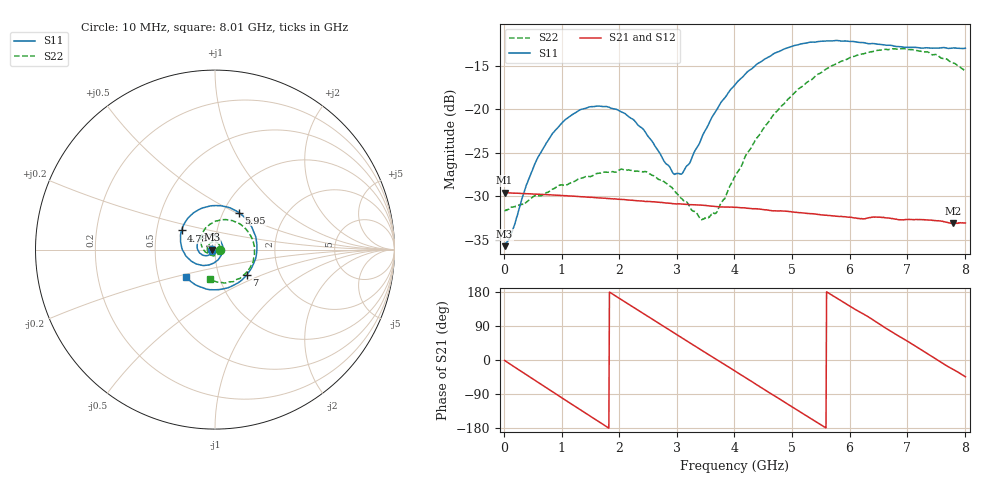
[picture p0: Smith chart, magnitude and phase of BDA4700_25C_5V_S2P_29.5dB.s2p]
!Agilent Technologies,E5071B,MY42404982,A.09.10
!Date: Mon Oct 20 13:41:26 2025
!Data & Calibration Information:
!Freq	S11:SOLT2(ON)	S21:SOLT2(ON)	S12:SOLT2(ON)	S22:SOLT2(ON)
# Hz S RI R 50
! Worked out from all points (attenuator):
!   801 points, 10 MHz to 8.01 GHz, reference 50 ohm
!   highest |S21| = -29.57 dB at 10 MHz (marker M1); lowest = -33.1 dB at 7.8 GHz (marker M2)
!   lowest |S11| = -35.7 dB at 10 MHz (marker M3), VSWR 1.03, Z = 48.4 - j0.113 ohm
!   |S11| at or under -10 dB: start of sweep to end of sweep
!   |S22| runs from -32.7 to -13.0 dB; largest |S21 - S12| = 0.0003
!   S11 on the Smith chart (normalised r, x): 10 MHz: 0.97, -0.00; 4.78 GHz: 0.67, +0.15; 5.95 GHz: 1.19, +0.52; 7 GHz: 1.37, -0.40; 8.01 GHz: 0.69, -0.22
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1e7  -0.0163 -0.00117  0.0332 -0.000676  0.0332 -0.000717  0.0262 -0.0008
1.4e8  -0.0176 -0.00937  0.032 -0.00815  0.032 -0.00817  0.0266 -0.00674
3.9e8  -0.0268 -0.0253  0.0254 -0.0207  0.0254 -0.0207  0.021 -0.0204
6.2e8  -0.0435 -0.0337  0.0153 -0.0287  0.0152 -0.0287  0.0115 -0.0297
1.01e9  -0.0804 -0.0235  -0.00579 -0.0315  -0.00583 -0.0314  -0.0152 -0.0335
1.35e9  -0.0995 0.00964  -0.0218 -0.0227  -0.0218 -0.0227  -0.036 -0.0179
2.08e9  -0.047 0.0827  -0.0275 0.0128  -0.0274 0.0128  -0.0299 0.0335
2.68e9  0.0313 0.0482  -0.00364 0.029  -0.00367 0.029  0.0126 0.0375
2.94e9  0.0421 0.00773  0.00866 0.0274  0.0087 0.0274  0.025 0.0242
3.09e9  0.0387 -0.0179  0.0151 0.0242  0.015 0.0243  0.0278 0.0126
3.42e9  0.00371 -0.0669  0.0251 0.0127  0.0251 0.0127  0.0198 -0.0121
3.54e9  -0.0162 -0.0787  0.0269 0.00737  0.027 0.00736  0.013 -0.02
3.7e9  -0.0492 -0.087  0.0276 0.000138  0.0276 4.01e-05  -0.000505 -0.0259
4.01e9  -0.1168 -0.0731  0.0239 -0.0133  0.0239 -0.0133  -0.032 -0.0257
4.78e9  -0.1861 0.1069  -0.00561 -0.0255  -0.00555 -0.0255  -0.0784 0.0639
5.35e9  -0.0662 0.2329  -0.0231 -0.00993  -0.0231 -0.00999  -0.0153 0.1476
5.95e9  0.1338 0.2059  -0.0202 0.0131  -0.0203 0.0131  0.1186 0.152
6.68e9  0.2303 -0.0307  0.00453 0.0233  0.00455 0.0233  0.2199 0.00056
7e9  0.1784 -0.1389  0.0149 0.0178  0.015 0.0178  0.2029 -0.085
7.42e9  0.0426 -0.2197  0.0228 0.00405  0.0227 0.00399  0.1228 -0.1648
7.8e9  -0.1008 -0.2004  0.02 -0.00932  0.02 -0.00929  0.0209 -0.1827
8.01e9  -0.1628 -0.153  0.0159 -0.0155  0.016 -0.0155  -0.03 -0.1626
